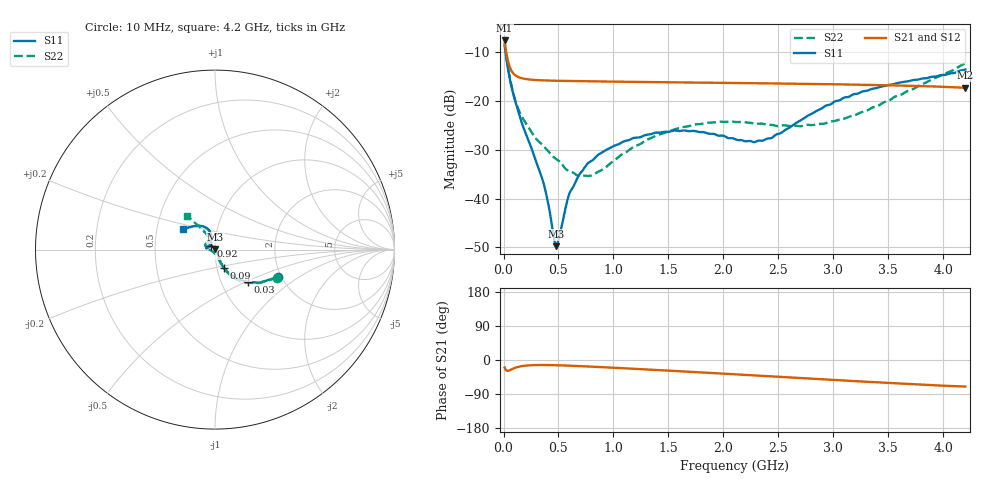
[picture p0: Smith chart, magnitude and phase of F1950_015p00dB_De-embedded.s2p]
! Integrated Device Technology
! Corporate Headquarters
! 6024 Silver Creek Valley Road
! San Jose, CA 95138  USA
! Phone:  1-408-284-8200
! Toll Free:  1-800-223-1366
! Webpage:  http://www.idt.com/
! Timing and RF Division
! 515 Groton Road, Suite 102
! Westford, MA 01886-6024
! Device:  F1950
! Description: 7-bit 0.25 dB Digital Step Attenuator
! Frequency:  150.0 -  4000.00 MHz
! Package:  4x4 mm Thin QFN Plastic Package: 24 pin
! Ports:  2 RF, 12 DC
!  Pin  1  = D0
!  Pin  2  = VDD
!  Pin  3  = Vmode
!  Pin  4  = GND
!  Pin  5  = RF1  =  Port 1
!  Pin  6  = GND
!  Pin  7  = GND
!  Pin  8  = GND
!  Pin  9  = GND
!  Pin 10  = GND
!  Pin 11  = GND
!  Pin 12  = GND
!  Pin 13  = GND
!  Pin 14  = RF2  =  Port 2
!  Pin 15  = GND
!  Pin 16  = LE
!  Pin 17  = CLK
!  Pin 18  = DATE
!  Pin 19  = D6
!  Pin 20  = D5
!  Pin 21  = D4
!  Pin 22  = D3
!  Pin 23  = D2
!  Pin 24  = D1
! State:  60
! Atten State:  15.00 dB
! Voltage:  +5.00 Volts
! Current:  Not Measured mA
! Data:  The device was measured on a the F195X evaluation board which has
!  individual transmission lines to the RF pins.  Data was collected
!  using a calibrated network analyzer.  The evaluation board was
!  de-embedded using a TRL calibration technique.
!  The reference plane is the edge of the package pin.
! Misc:  Board 2019
!  Action Tracker AT0250
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# GHz S dB R 50
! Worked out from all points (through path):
!   420 points, 10 MHz to 4.2 GHz, reference 50 ohm
!   highest |S21| = -7.56 dB at 10 MHz (marker M1); lowest = -17.3 dB at 4.2 GHz (marker M2)
!   group delay of S21, straight-line fit = 40.6 ps
!   lowest |S11| = -49.7 dB at 480 MHz (marker M3), VSWR 1.01, Z = 50.3 + j0.199 ohm
!   |S11| at or under -10 dB: 18.94 MHz to end of sweep
!   |S22| runs from -35.4 to -8.4 dB; largest |S21 - S12| = 0.00024
!   S11 on the Smith chart (normalised r, x): 10 MHz: 1.91, -0.68; 30 MHz: 1.33, -0.52; 90 MHz: 1.08, -0.23; 920 MHz: 0.95, +0.04; 4.2 GHz: 0.68, +0.17
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0.01  -8.39 -23.7  -7.56 -19.8  -7.56 -19.8  -8.39 -24.4
0.03  -11.79 -44.7  -10.64 -28.3  -10.64 -28.3  -11.70 -45.6
0.05  -14.59 -54.8  -12.56 -27.9  -12.56 -27.9  -14.35 -56.0
0.09  -18.68 -63.8  -14.35 -22.4  -14.35 -22.4  -18.53 -63.5
0.18  -25.34 -64.0  -15.38 -15.6  -15.38 -15.6  -23.69 -69.5
0.36  -36.51 -47.8  -15.75 -13.2  -15.75 -13.2  -29.12 -75.0
0.4  -40.28 -40.4  -15.78 -13.3  -15.78 -13.3  -30.09 -75.6
0.46  -48.32 0.1  -15.82 -13.6  -15.82 -13.6  -31.56 -81.4
0.48  -49.74 37.5  -15.83 -13.8  -15.83 -13.8  -31.89 -83.8
0.5  -48.41 71.3  -15.84 -14.0  -15.84 -14.0  -32.20 -85.3
0.6  -38.91 117.7  -15.88 -15.0  -15.88 -15.0  -34.33 -99.0
0.71  -34.48 128.7  -15.91 -16.3  -15.91 -16.3  -35.31 -118.5
0.92  -30.18 141.9  -15.98 -19.2  -15.98 -19.3  -33.77 -158.7
1.17  -27.66 154.2  -16.05 -22.9  -16.05 -22.9  -29.54 178.2
1.41  -26.46 164.6  -16.12 -26.6  -16.12 -26.6  -26.88 168.4
1.73  -26.11 171.4  -16.19 -31.7  -16.19 -31.7  -24.84 159.5
2.11  -27.85 161.4  -16.29 -37.9  -16.29 -37.9  -24.29 150.1
2.43  -27.62 127.0  -16.38 -43.0  -16.38 -43.0  -24.86 140.3
2.81  -22.51 104.9  -16.48 -49.4  -16.48 -49.4  -24.92 125.1
3.19  -18.56 108.6  -16.62 -55.7  -16.62 -55.7  -22.92 118.3
3.51  -16.65 117.8  -16.76 -60.7  -16.76 -60.8  -19.83 119.4
4.2  -13.52 146.8  -17.26 -70.1  -17.26 -70.2  -12.25 130.0
